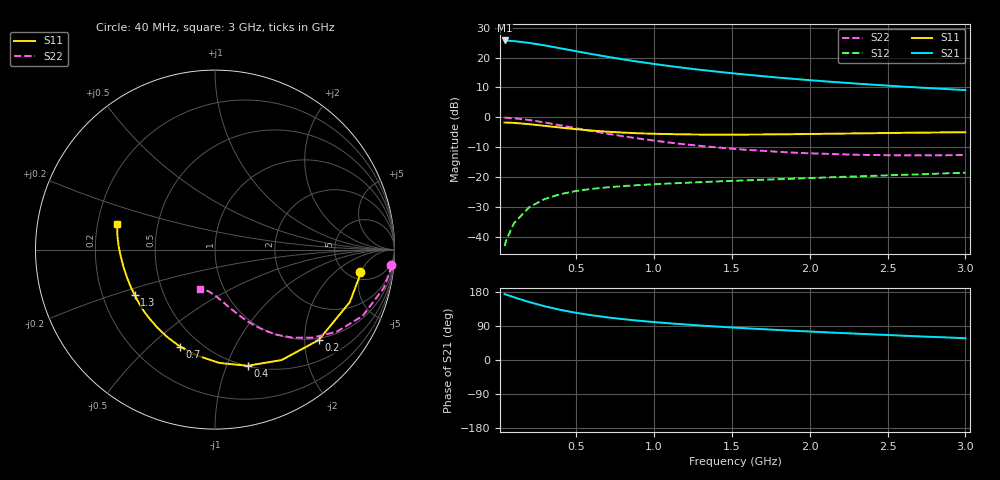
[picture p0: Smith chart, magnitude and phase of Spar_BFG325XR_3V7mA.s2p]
! Filename: 37BFG325XR.s2p
! Title: BFG325XR,RN20042071,Lot:TT3899C,B:Y13641,Sl.:1
! Bias: VCE=2.999V; IC=6.939mA;
! Company: NXP Semiconductors NL
! User: Q&R DSC-N
! Measure time: 29 Mar 2004 / 13:39:02
#  MHz  S  MA  R 50
! Freq  S11  S21  S12  S22  :
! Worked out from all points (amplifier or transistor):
!   32 points, 40 MHz to 3 GHz, reference 50 ohm
!   highest |S21| = 25.8 dB at 40 MHz (marker M1)
!   |S21| within 3 dB of that: start of sweep to 437.4 MHz
!   unconditionally stable (mu >= 1): 2.572 GHz to end of sweep
!   at 400 MHz: K = 0.27, MSG = 24.4 dB, |S12| = -25.7 dB
!   at 1.5 GHz: K = 0.79, MSG = 18.0 dB, |S12| = -21.3 dB
!   at 3 GHz: K = 1.03, MAG = 12.8 dB, |S12| = -18.6 dB
!   S11 on the Smith chart (normalised r, x): 40 MHz: 6.43, -4.78; 200 MHz: 0.95, -2.33; 400 MHz: 0.50, -1.19; 700 MHz: 0.39, -0.63; 1.3 GHz: 0.34, -0.24; 3 GHz: 0.28, +0.12
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40  0.8188 -8.6  19.4 173.9  0.006939 85.4  0.9864 -5.1
50  0.8179 -10.8  19.32 172.5  0.008617 84.2  0.9843 -6.4
100  0.806 -21.3  18.92 165.6  0.01686 78.7  0.965 -12.7
200  0.7667 -41.1  17.61 152.6  0.0315 68.8  0.9011 -24.3
300  0.7187 -58.9  15.99 141.5  0.04307 60.8  0.8179 -34.0
400  0.6722 -74.3  14.32 132.2  0.05179 54.5  0.7325 -42.0
500  0.6319 -87.9  12.8 124.5  0.05837 49.9  0.6554 -48.5
600  0.5992 -99.6  11.48 118.0  0.06328 46.4  0.5886 -53.8
700  0.5745 -109.8  10.34 112.5  0.06718 43.9  0.5312 -58.2
800  0.5552 -118.6  9.363 107.8  0.07044 42.0  0.4827 -62.0
900  0.5403 -126.5  8.537 103.7  0.07314 40.7  0.442 -65.4
1000  0.53 -133.6  7.834 100.0  0.07559 39.7  0.4077 -68.2
1100  0.5237 -139.8  7.228 96.7  0.07791 39.1  0.3773 -71.0
1200  0.5176 -145.4  6.697 93.8  0.08 38.7  0.3521 -73.7
1300  0.514 -150.4  6.239 90.9  0.08209 38.4  0.3318 -76.2
1400  0.5134 -155.1  5.844 88.3  0.08425 38.3  0.3139 -78.5
1600  0.5143 -163.0  5.169 83.5  0.08798 38.3  0.2844 -83.2
1800  0.5194 -169.8  4.624 79.2  0.09195 38.6  0.2642 -87.5
2100  0.5298 -178.0  4.001 73.1  0.09806 39.0  0.2448 -94.1
2300  0.5382 177.5  3.673 69.5  0.1024 39.5  0.2359 -98.2
2600  0.5498 171.6  3.269 64.2  0.109 40.0  0.2307 -104.0
3000  0.5623 165.0  2.863 57.4  0.1179 40.1  0.2329 -111.2
